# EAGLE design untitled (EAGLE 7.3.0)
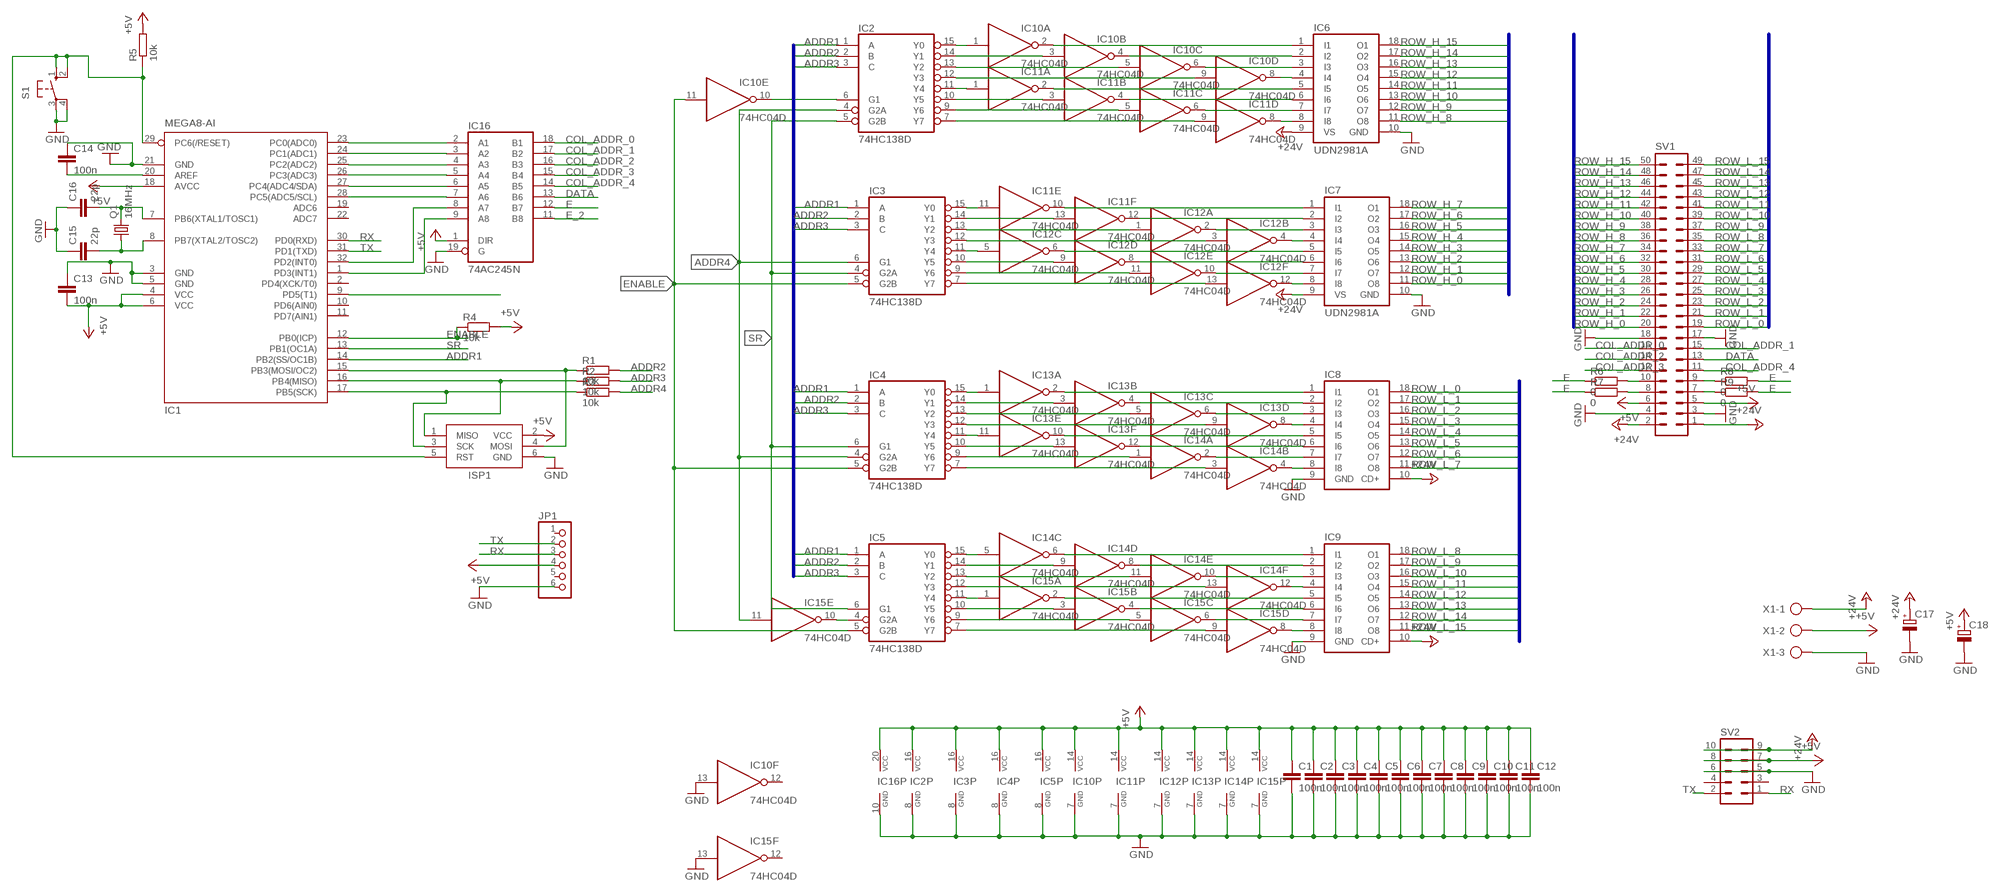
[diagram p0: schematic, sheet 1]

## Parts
C1  100n  C-EUC0805  [C0805]
C2  100n  C-EUC0805  [C0805]
C3  100n  C-EUC0805  [C0805]
C4  100n  C-EUC0805  [C0805]
C5  100n  C-EUC0805  [C0805]
C6  100n  C-EUC0805  [C0805]
C7  100n  C-EUC0805  [C0805]
C8  100n  C-EUC0805  [C0805]
C9  100n  C-EUC0805  [C0805]
C10  100n  C-EUC0805  [C0805]
C11  100n  C-EUC0805  [C0805]
C12  100n  C-EUC0805  [C0805]
C13  100n  C-EUC0805  [C0805]
C14  100n  C-EUC0805  [C0805]
C15  22p  C-EUC0805  [C0805]
C16  22p  C-EUC0805  [C0805]
C17  CPOL-EUTT5D7L  [TT5D7L]
C18  CPOL-EUTT2D7  [TT2D7]
IC1  MEGA8-AI  [TQFP32-08]
IC2  74HC138D  [SO16]
IC3  74HC138D  [SO16]
IC4  74HC138D  [SO16]
IC5  74HC138D  [SO16]
IC6  UDN2981A  [DIL18]
IC7  UDN2981A  [DIL18]
IC8  ULN2803A  [DIL18]
IC9  ULN2803A  [DIL18]
IC10  74HC04D  [SO14]
IC11  74HC04D  [SO14]
IC12  74HC04D  [SO14]
IC13  74HC04D  [SO14]
IC14  74HC04D  [SO14]
IC15  74HC04D  [SO14]
IC16  74AC245N  [DIL20]
ISP1  AVRISP-6  [AVRISP]
JP1  PINHD-1X6CB  [1X06-CLEANBIG]
Q1  16MHz  CRYSTALHC49UP  [HC49UP]
R1  10k  R-EU_R1206  [R1206]
R2  10k  R-EU_R1206  [R1206]
R3  10k  R-EU_R1206  [R1206]
R4  10k  R-EU_R1206  [R1206]
R5  10k  R-EU_R1206  [R1206]
R6  0  R-EU_M0805  [M0805]
R7  0  R-EU_M0805  [M0805]
R8  0  R-EU_M0805  [M0805]
R9  0  R-EU_M0805  [M0805]
S1  10-XX  [B3F-10XX]
SV1  ML50  [ML50]
SV2  ML10  [ML10]
X1  AK300/3  [AK300/3]

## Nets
+5V: C1.1 C2.1 C3.1 C4.1 C5.1 C6.1 C7.1 C8.1 C9.1 C10.1 C11.1 C12.1 C13.2 C18.+ IC1.4(VCC) IC1.6(VCC) IC1.18(AVCC) IC2.16(VCC) IC3.16(VCC) IC4.16(VCC) IC5.16(VCC) IC10.14(P:VCC) IC11.14(P:VCC) IC12.14(P:VCC) IC13.14(P:VCC) IC14.14(P:VCC) IC15.14(P:VCC) IC16.1(DIR) IC16.20(VCC) ISP1.2(VCC) JP1.4 R4.2 R5.2 SV1.5 SV1.6 SV2.7 SV2.8 X1.2
+24V: C17.+ IC6.9(VS) IC7.9(VS) IC8.10(CD+) IC9.10(CD+) SV1.1 SV1.2 SV2.9 SV2.10 X1.1
ADDR1: IC1.14(PB2(SS/OC1B)) IC2.1(A) IC3.1(A) IC4.1(A) IC5.1(A)
ADDR2: IC2.2(B) IC3.2(B) IC4.2(B) IC5.2(B) R1.2
ADDR3: IC2.3(C) IC3.3(C) IC4.3(C) IC5.3(C) R2.2
ADDR4: IC2.4(G2A) IC3.6(G1) IC4.4(G2A) IC15.11(E:I) R3.2
COL_ADDR_0: IC16.18(B1) SV1.16
COL_ADDR_1: IC16.17(B2) SV1.15
COL_ADDR_2: IC16.16(B3) SV1.14
COL_ADDR_3: IC16.15(B4) SV1.12
COL_ADDR_4: IC16.14(B5) SV1.11
DATA: IC16.13(B6) SV1.13
E: IC16.12(B7) R6.1 R7.1 R8.2 R9.2
E_2: IC16.11(B8)
ENABLE: IC1.12(PB0(ICP)) IC3.5(G2B) IC4.5(G2B) IC5.5(G2B) IC10.11(E:I) R4.1
GND: C1.2 C2.2 C3.2 C4.2 C5.2 C6.2 C7.2 C8.2 C9.2 C10.2 C11.2 C12.2 C13.1 C14.1 C15.1 C16.1 C17.- C18.- IC1.3(GND) IC1.5(GND) IC1.21(GND) IC2.8(GND) IC3.8(GND) IC4.8(GND) IC5.8(GND) IC6.10(GND) IC7.10(GND) IC8.9(GND) IC9.9(GND) IC10.7(P:GND) IC10.13(F:I) IC11.7(P:GND) IC12.7(P:GND) IC13.7(P:GND) IC14.7(P:GND) IC15.7(P:GND) IC15.13(F:I) IC16.10(GND) IC16.19(G) ISP1.6(GND) JP1.6 S1.3(P) S1.4(P1) SV1.3 SV1.4 SV1.17 SV1.18 SV2.5 SV2.6 X1.3
N$1: IC9.8(I8) IC15.8(D:O)
N$2: IC9.7(I7) IC15.6(C:O)
N$3: IC9.6(I6) IC15.4(B:O)
N$4: IC6.1(I1) IC10.2(A:O)
N$5: IC6.2(I2) IC10.4(B:O)
N$6: IC6.3(I3) IC10.6(C:O)
N$7: IC2.15(Y0) IC10.1(A:I)
N$8: IC2.14(Y1) IC10.3(B:I)
N$9: IC2.13(Y2) IC10.5(C:I)
N$10: IC5.10(Y5) IC15.3(B:I)
N$11: IC5.9(Y6) IC15.5(C:I)
N$12: IC5.7(Y7) IC15.9(D:I)
N$13: IC6.8(I8) IC11.8(D:O)
N$14: IC2.12(Y3) IC10.9(D:I)
N$15: IC2.11(Y4) IC11.1(A:I)
N$16: IC2.10(Y5) IC11.3(B:I)
N$17: IC2.9(Y6) IC11.5(C:I)
N$18: IC2.7(Y7) IC11.9(D:I)
N$19: IC6.7(I7) IC11.6(C:O)
N$20: IC6.6(I6) IC11.4(B:O)
N$21: IC6.5(I5) IC11.2(A:O)
N$22: IC6.4(I4) IC10.8(D:O)
N$23: IC7.1(I1) IC11.10(E:O)
N$24: IC7.2(I2) IC11.12(F:O)
N$25: IC7.3(I3) IC12.2(A:O)
N$26: IC3.15(Y0) IC11.11(E:I)
N$27: IC3.14(Y1) IC11.13(F:I)
N$28: IC3.13(Y2) IC12.1(A:I)
N$29: IC8.1(I1) IC13.2(A:O)
N$30: IC3.12(Y3) IC12.3(B:I)
N$31: IC3.11(Y4) IC12.5(C:I)
N$32: IC3.10(Y5) IC12.9(D:I)
N$33: IC3.9(Y6) IC12.11(E:I)
N$34: IC3.7(Y7) IC12.13(F:I)
N$35: IC7.7(I7) IC12.10(E:O)
N$36: IC7.6(I6) IC12.8(D:O)
N$37: IC7.5(I5) IC12.6(C:O)
N$38: IC8.2(I2) IC13.4(B:O)
N$39: IC8.3(I3) IC13.6(C:O)
N$40: IC4.15(Y0) IC13.1(A:I)
N$41: IC4.14(Y1) IC13.3(B:I)
N$42: IC4.13(Y2) IC13.5(C:I)
N$43: IC4.12(Y3) IC13.9(D:I)
N$44: IC4.11(Y4) IC13.11(E:I)
N$45: IC4.10(Y5) IC13.13(F:I)
N$46: IC4.9(Y6) IC14.1(A:I)
N$47: IC4.7(Y7) IC14.3(B:I)
N$48: IC8.7(I7) IC14.2(A:O)
N$49: IC8.6(I6) IC13.12(F:O)
N$50: IC8.5(I5) IC13.10(E:O)
N$51: IC7.4(I4) IC12.4(B:O)
N$52: IC7.8(I8) IC12.12(F:O)
N$53: IC8.4(I4) IC13.8(D:O)
N$54: IC8.8(I8) IC14.4(B:O)
N$55: IC5.11(Y4) IC15.1(A:I)
N$56: IC9.5(I5) IC15.2(A:O)
N$57: IC9.4(I4) IC14.12(F:O)
N$58: IC5.12(Y3) IC14.13(F:I)
N$59: IC5.13(Y2) IC14.11(E:I)
N$60: IC9.3(I3) IC14.10(E:O)
N$61: IC9.2(I2) IC14.8(D:O)
N$62: IC5.14(Y1) IC14.9(D:I)
N$63: IC5.15(Y0) IC14.5(C:I)
N$64: IC9.1(I1) IC14.6(C:O)
N$65: IC5.4(G2A) IC15.10(E:O)
N$66: IC1.15(PB3(MOSI/OC2)) ISP1.4(MOSI) R1.1
N$67: IC1.1(PD3(INT1)) IC16.9(A8)
N$69: IC1.16(PB4(MISO)) ISP1.1(MISO) R2.1
N$70: IC1.17(PB5(SCK)) ISP1.3(SCK) R3.1
N$71: IC1.32(PD2(INT0)) IC16.8(A7)
N$72: IC2.6(G1) IC10.10(E:O)
N$74: R6.2 SV1.10
N$75: IC1.9(PD5(T1))
N$76: IC1.23(PC0(ADC0)) IC16.2(A1)
N$77: IC1.24(PC1(ADC1)) IC16.3(A2)
N$78: IC1.25(PC2(ADC2)) IC16.4(A3)
N$79: IC1.26(PC3(ADC3)) IC16.5(A4)
N$80: IC1.27(PC4(ADC4/SDA)) IC16.6(A5)
N$81: IC1.28(PC5(ADC5/SCL)) IC16.7(A6)
N$82: C14.2 IC1.20(AREF)
N$83: IC1.29(PC6(/RESET)) ISP1.5(RST) R5.1 S1.1(S) S1.2(S1)
N$84: C16.2 IC1.7(PB6(XTAL1/TOSC1)) Q1.2
N$85: C15.2 IC1.8(PB7(XTAL2/TOSC2)) Q1.1
N$86: R7.2 SV1.8
N$87: R8.1 SV1.9
N$88: R9.1 SV1.7
ROW_H_0: IC7.11(O8) SV1.20
ROW_H_1: IC7.12(O7) SV1.22
ROW_H_2: IC7.13(O6) SV1.24
ROW_H_3: IC7.14(O5) SV1.26
ROW_H_4: IC7.15(O4) SV1.28
ROW_H_5: IC7.16(O3) SV1.30
ROW_H_6: IC7.17(O2) SV1.32
ROW_H_7: IC7.18(O1) SV1.34
ROW_H_8: IC6.11(O8) SV1.36
ROW_H_9: IC6.12(O7) SV1.38
ROW_H_10: IC6.13(O6) SV1.40
ROW_H_11: IC6.14(O5) SV1.42
ROW_H_12: IC6.15(O4) SV1.44
ROW_H_13: IC6.16(O3) SV1.46
ROW_H_14: IC6.17(O2) SV1.48
ROW_H_15: IC6.18(O1) SV1.50
ROW_L_0: IC8.18(O1) SV1.19
ROW_L_1: IC8.17(O2) SV1.21
ROW_L_2: IC8.16(O3) SV1.23
ROW_L_3: IC8.15(O4) SV1.25
ROW_L_4: IC8.14(O5) SV1.27
ROW_L_5: IC8.13(O6) SV1.29
ROW_L_6: IC8.12(O7) SV1.31
ROW_L_7: IC8.11(O8) SV1.33
ROW_L_8: IC9.18(O1) SV1.35
ROW_L_9: IC9.17(O2) SV1.37
ROW_L_10: IC9.16(O3) SV1.39
ROW_L_11: IC9.15(O4) SV1.41
ROW_L_12: IC9.14(O5) SV1.43
ROW_L_13: IC9.13(O6) SV1.45
ROW_L_14: IC9.12(O7) SV1.47
ROW_L_15: IC9.11(O8) SV1.49
RX: IC1.30(PD0(RXD)) JP1.3 SV2.1
SR: IC1.13(PB1(OC1A)) IC2.5(G2B) IC3.4(G2A) IC4.6(G1) IC5.6(G1)
TX: IC1.31(PD1(TXD)) JP1.2 SV2.2
Unconnected: IC1.2(PD4(XCK/T0)) IC1.10(PD6(AIN0)) IC1.11(PD7(AIN1)) IC1.19(ADC6) IC1.22(ADC7) IC10.12(F:O) IC15.12(F:O) JP1.1 JP1.5 SV2.3 SV2.4

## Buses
ROW_H_[0..15]
ROW_L_[0..15]
ADDR[1..3]

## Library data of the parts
C1-C16 = rcl:C-EU: CAPACITOR, European symbol
C17 C18 = rcl:CPOL-EU: POLARIZED CAPACITOR, European symbol
IC1 = atmel:MEGA8: MICROCONTROLLER 8 Kbytes FLASH, 1 kbytes SRAM, 512 bytes EEPROM, USART, 6-channel 10 bit ADC, 2-channel 8 bit ADC Pin compatible with Atmega48, ATMega88, ATMega168 Source: avr.lbr; MPN: ATMEGA8-16AU; OC_FARNELL: 9171371; OC_NEWARK: 73M8863
IC2-IC5 = 74xx-eu:74*138: 3-line to 8-line DECODER/DEMULTIPLEXER
IC6 IC7 = uln-udn:UDN298*: DRIVER ARRAY Source: Allegro Microsystems Inc. / UDN2981-UDN2984.pdf
IC8 IC9 = uln-udn:ULN2803A: DRIVER ARRAY
IC10-IC15 = 74xx-eu:74*04: Hex INVERTER
IC16 = 74xx-eu:74*245: Octal BUS TRANSCEIVER, 3-state
ISP1 = adafruit:AVRISP: AVR ISP HEADER Standard 6 pin header for AVR programming
JP1 = adafruit:PINHD-1X6: PIN HEADER
Q1 = crystal:CRYSTAL: CRYSTAL; OC_FARNELL: unknown; OC_NEWARK: unknown
R1-R9 = rcl:R-EU_: RESISTOR, European symbol
S1 = switch-omron:10-XX: OMRON SWITCH; MPN: B3F-1000; OC_FARNELL: 176432; OC_NEWARK: 36M3542
SV1 = con-harting-ml:ML50: HARTING; OC_FARNELL: unknown; OC_NEWARK: unknown
SV2 = con-harting-ml:ML10: HARTING; OC_FARNELL: unknown; OC_NEWARK: unknown
X1 = con-ptr500:AK300/3: CONNECTOR; OC_FARNELL: unknown; OC_NEWARK: unknown

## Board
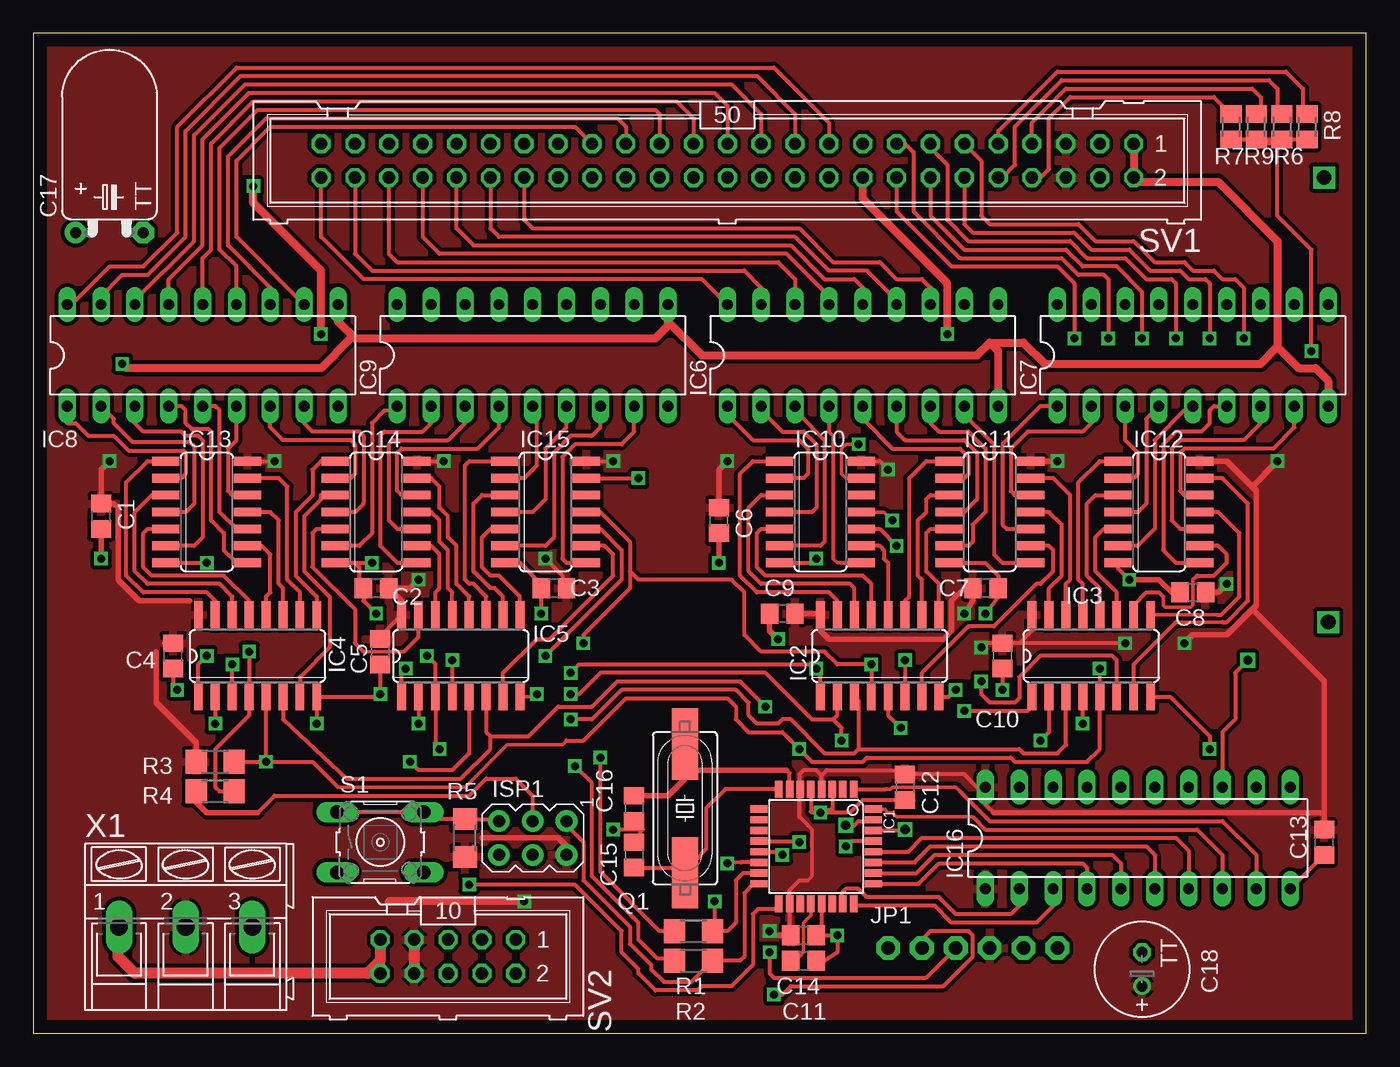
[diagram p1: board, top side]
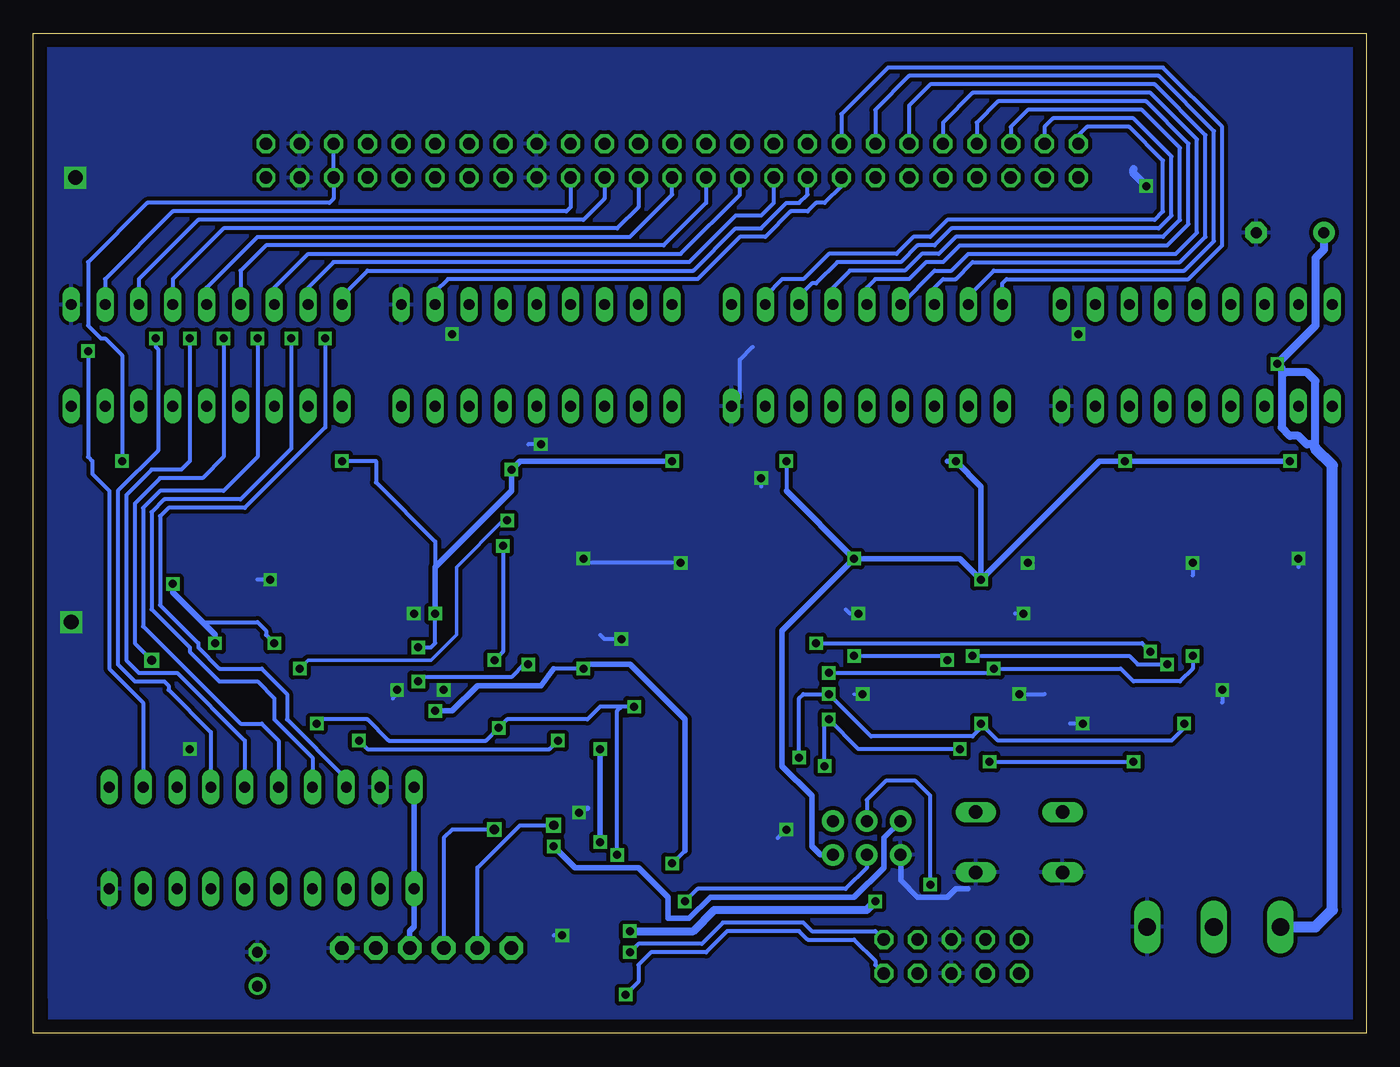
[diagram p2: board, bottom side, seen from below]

Size 100 x 75 mm. Coordinates in mm from the lower left corner, seen from the top.
Outline: 0,0 100,0 100,75 0,75 0,0
Copper layers (1*16): Top 0.035mm / dielectric 1.5mm / Bottom 0.035mm
Design rules "default *": minimum track width 6mil, minimum drill 10mil, track to track 8mil, track to pad 8mil, pad to pad 8mil, via to via 8mil, smd to smd 8mil, copper to edge 40mil, drill to drill 8mil, minimum pad ring 10mil, minimum via ring 8mil, stop-mask expansion 4mil, vias tented up to drill 0mil, thermal gap 10mil

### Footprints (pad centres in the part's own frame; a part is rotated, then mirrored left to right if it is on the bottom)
C0805 = smd 1.3 x 1.5: 1 -0.95,0; 2 0.95,0
TT5D7L = drill 0.813 pad 1.6: + -2.54,0 | drill 0.813 pad 1.6 octagon: - 2.54,0
TT2D7 = drill 0.813: + -1.27,0 | drill 0.813 octagon: - 1.27,0
TQFP32-08 = smd 1.27 x 0.559: 1 -4.293,2.8; 2 -4.293,2; 3 -4.293,1.2; 4 -4.293,0.4; 5 -4.293,-0.4; 6 -4.293,-1.2; 7 -4.293,-2; 8 -4.293,-2.8; 17 4.293,-2.8; 18 4.293,-2; 19 4.293,-1.2; 20 4.293,-0.4; 21 4.293,0.4; 22 4.293,1.2; 23 4.293,2; 24 4.293,2.8 | smd 0.559 x 1.27: 9 -2.8,-4.293; 10 -2,-4.293; 11 -1.2,-4.293; 12 -0.4,-4.293; 13 0.4,-4.293; 14 1.2,-4.293; 15 2,-4.293; 16 2.8,-4.293; 25 2.8,4.293; 26 2,4.293; 27 1.2,4.293; 28 0.4,4.293; 29 -0.4,4.293; 30 -1.2,4.293; 31 -2,4.293; 32 -2.8,4.293
SO16 = smd 0.66 x 2.032: 1 -4.445,-3.073; 2 -3.175,-3.073; 3 -1.905,-3.073; 4 -0.635,-3.073; 5 0.635,-3.073; 6 1.905,-3.073; 7 3.175,-3.073; 8 4.445,-3.073; 9 4.445,3.073; 10 3.175,3.073; 11 1.905,3.073; 12 0.635,3.073; 13 -0.635,3.073; 14 -1.905,3.073; 15 -3.175,3.073; 16 -4.445,3.073
DIL18 = drill 0.813 long: 1 -10.16,-3.81; 2 -7.62,-3.81; 3 -5.08,-3.81; 4 -2.54,-3.81; 5 0,-3.81; 6 2.54,-3.81; 7 5.08,-3.81; 8 7.62,-3.81; 9 10.16,-3.81; 10 10.16,3.81; 11 7.62,3.81; 12 5.08,3.81; 13 2.54,3.81; 14 0,3.81; 15 -2.54,3.81; 16 -5.08,3.81; 17 -7.62,3.81; 18 -10.16,3.81
SO14 = smd 0.66 x 2.032: 1 -3.81,-3.073; 2 -2.54,-3.073; 3 -1.27,-3.073; 4 0,-3.073; 5 1.27,-3.073; 6 2.54,-3.073; 7 3.81,-3.073; 8 3.81,3.073; 9 2.54,3.073; 10 1.27,3.073; 11 0,3.073; 12 -1.27,3.073; 13 -2.54,3.073; 14 -3.81,3.073
DIL20 = drill 0.813 long: 1 -11.43,-3.81; 2 -8.89,-3.81; 3 -6.35,-3.81; 4 -3.81,-3.81; 5 -1.27,-3.81; 6 1.27,-3.81; 7 3.81,-3.81; 8 6.35,-3.81; 9 8.89,-3.81; 10 11.43,-3.81; 11 11.43,3.81; 12 8.89,3.81; 13 6.35,3.81; 14 3.81,3.81; 15 1.27,3.81; 16 -1.27,3.81; 17 -3.81,3.81; 18 -6.35,3.81; 19 -8.89,3.81; 20 -11.43,3.81
AVRISP = drill 0.9 pad 1.626: 1 -1.27,2.54; 2 1.27,2.54; 3 -1.27,0; 4 1.27,0; 5 -1.27,-2.54; 6 1.27,-2.54
1X06-CLEANBIG = drill 1.016 pad 1.778 octagon: 1 -6.35,0; 2 -3.81,0; 3 -1.27,0; 4 1.27,0; 5 3.81,0; 6 6.35,0
HC49UP = smd 5.334 x 1.93: 1 -4.826,0; 2 4.826,0
R1206 = smd 1.6 x 1.803: 1 -1.422,0; 2 1.422,0
M0805 = smd 1.3 x 1.6: 1 -0.95,0; 2 0.95,0
B3F-10XX = drill 1.016 long: 1 -3.251,2.261; 2 3.251,2.261; 3 -3.251,-2.261; 4 3.251,-2.261
ML50 = drill 0.914 octagon: 1 -30.48,-1.27; 2 -30.48,1.27; 3 -27.94,-1.27; 4 -27.94,1.27; 5 -25.4,-1.27; 6 -25.4,1.27; 7 -22.86,-1.27; 8 -22.86,1.27; 9 -20.32,-1.27; 10 -20.32,1.27; 11 -17.78,-1.27; 12 -17.78,1.27; 13 -15.24,-1.27; 14 -15.24,1.27; 15 -12.7,-1.27; 16 -12.7,1.27; 17 -10.16,-1.27; 18 -10.16,1.27; 19 -7.62,-1.27; 20 -7.62,1.27; 21 -5.08,-1.27; 22 -5.08,1.27; 23 -2.54,-1.27; 24 -2.54,1.27; 25 0,-1.27; 26 0,1.27; 27 2.54,-1.27; 28 2.54,1.27; 29 5.08,-1.27; 30 5.08,1.27; 31 7.62,-1.27; 32 7.62,1.27; 33 10.16,-1.27; 34 10.16,1.27; 35 12.7,-1.27; 36 12.7,1.27; 37 15.24,-1.27; 38 15.24,1.27; 39 17.78,-1.27; 40 17.78,1.27; 41 20.32,-1.27; 42 20.32,1.27; 43 22.86,-1.27; 44 22.86,1.27; 45 25.4,-1.27; 46 25.4,1.27; 47 27.94,-1.27; 48 27.94,1.27; 49 30.48,-1.27; 50 30.48,1.27
ML10 = drill 0.914 octagon: 1 -5.08,-1.27; 2 -5.08,1.27; 3 -2.54,-1.27; 4 -2.54,1.27; 5 0,-1.27; 6 0,1.27; 7 2.54,-1.27; 8 2.54,1.27; 9 5.08,-1.27; 10 5.08,1.27
AK300/3 = drill 1.321 long: 1 -5.004,0; 2 0,0; 3 5.004,0

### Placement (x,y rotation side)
C1  5.08,38.78 270 top
C2  25.72,33.38 180 top
C3  39.05,33.38 180 top
C4  10.48,28.3 270 top
C5  26.04,28.62 270 top
C6  51.44,38.47 270 top
C7  71.44,33.38 0 top
C8  87,33.07 180 top
C9  56.2,31.48 180 top
C10  72.71,28.3 270 top
C11  57.78,7.35 0 top
C12  65.41,18.46 270 top
C13  96.84,14.34 90 top
C14  57.78,5.45 180 top
C15  45.09,13.38 270 top
C16  45.09,16.88 90 top
C17  5.71,60.05 0 top
C18  83.19,4.81 90 top
IC1  58.74,14.02 270 top
IC2  63.5,28.3 0 top
IC3  79.38,28.3 0 top
IC4  16.83,28.3 0 top
IC5  32.07,28.3 0 top
IC6  62.23,50.85 0 top
IC7  87,50.85 0 top
IC8  12.7,50.85 0 top
IC9  37.47,50.85 0 top
IC10  59.05,39.1 270 top
IC11  71.75,39.1 270 top
IC12  84.45,39.1 270 top
IC13  13.02,39.1 270 top
IC14  25.72,39.1 270 top
IC15  38.42,39.1 270 top
IC16  82.87,14.65 0 top
ISP1  37.47,14.65 270 top
JP1  70.48,6.4 0 top
Q1  48.9,16.88 90 top
R1  49.53,7.67 180 top
R2  49.53,5.45 180 top
R3  13.65,18.14 0 top
R4  13.65,20.37 180 top
R5  32.38,14.65 270 top
R6  93.66,67.99 90 top
R7  89.85,67.99 90 top
R8  95.57,67.99 270 top
R9  91.76,67.99 270 top
S1  26.04,14.34 0 top
SV1  52.07,65.45 180 top
SV2  31.11,5.76 180 top
X1  11.43,7.99 0 top

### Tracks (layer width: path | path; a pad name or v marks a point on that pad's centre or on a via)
+5V  (via drill 0.6)
  Top 0.254: 58.1,15.61 58.42,15.29 58.42,11.79 58.1,11.48
  Top 0.305: IC13.14 v18.1,42.91 | IC14.14 v30.8,42.91 | 70.49,32.44 C7.1 69.85,33.38 | 73.98,29.26 73.03,29.26 | 73.03,29.26 C10.1 | IC3.16 74.93,30.21 73.98,29.26 | 73.03,29.26 71.44,29.26 v71.12,28.94 | IC10.14 63.5,42.91 v64.14,42.27 | IC15.14 v43.5,42.91 | v38.42,35.61 39.69,34.34 39.69,33.7 C3.1 | C5.1 26.04,29.79 IC5.16 | IC4.16 12.38,31.8 | v81.92,29.26 73.98,29.26 | 58.95,31.48 IC2.16 | 72.07,16.56 71.44,17.19 IC16.20 70.8,18.46 69.85,19.41 C12.1 | 96.52,16.56 96.84,16.24 | IC1.4 59.14,19.33 | 59.14,19.33 58.74,19.73 57.78,19.73 57.47,19.41 57.47,18.38 IC1.6 57.47,18.24 57.47,16.24 58.1,15.61 | C12.1 65.09,19.09 | 59.14,19.33 59.54,19.73 65.08,19.73 C12.1 | C11.1 56.74,7.76 IC1.18 56.74,10.75 57.47,11.48 58.1,11.48 | R5.2 32.38,13.38 33.02,14.02 | 65.41,19.1 C12.1 | 56.83,7.03 57.15,7.35
  Top 0.406: 70.49,32.44 v69.85,31.48 | C8.1 88.9,33.07 v89.53,33.7 | IC2.16 59.05,30.21 59.69,29.57 68.26,29.57 68.9,30.21 68.9,32.43 69.85,33.38 | C6.1 51.44,42.27 v52.07,42.91 | IC5.16 27.62,32.43 C2.1 28.26,33.38 v28.89,34.02 | v5.71,42.91 5.08,42.27 C1.1 5.4,39.73 6.03,39.73 6.35,39.42 6.35,34.02 7.94,32.43 11.75,32.43 | IC11.14 v76.83,42.91 | C9.1 58.95,31.48 | 91.44,41.01 89.53,42.91 IC12.14 | 91.44,41.01 91.76,40.69 91.76,32.11 91.44,31.8 | 91.44,31.8 89.53,29.89 87,29.89 v86.36,29.26 | v93.34,42.91 91.44,41.01 | C13.2 96.84,16.24 96.84,26.4 91.44,31.8 | 72.07,16.56 96.52,16.56 | R4.2 12.23,21.79 9.21,24.81 9.21,28.62 | 9.84,29.26 C4.1 | 33.66,14.65 39.37,14.65 40.01,14.02 ISP1.2 | 57.15,7.35 55.56,7.35 v55.24,7.67
  Top 0.61: v36.83,9.89 26.67,9.89
  Top 0.813: SV2.7 SV2.8
  Bottom 0.305: v71.12,28.94 70.17,28.94 69.85,29.26 v69.85,31.48 | v89.53,33.7 89.53,33.07 | v43.5,42.91 43.5,40.69 | 69.85,34.97 69.85,36.88 74.3,41.32 74.3,42.91 v76.83,42.91 | 87.31,30.84 83.19,30.84 82.55,30.21 82.55,29.89 v81.92,29.26 | SV1.5 SV1.6 77.47,62.59 77.79,62.28 91.44,62.28 95.89,57.83 95.89,53.07 94.93,52.12 94.61,52.12 93.34,50.85 v93.34,42.91 | v38.42,35.61 39.69,34.34
  Bottom 0.406: 31.43,42.91 v30.8,42.91 28.89,41.01 v28.89,34.02 | v69.85,31.48 69.85,34.97 64.14,40.69 v64.14,42.27 63.5,42.91 v52.07,42.91 | 43.5,40.69 v38.42,35.61 | v5.71,42.91 v18.1,42.91 20,42.91 v28.89,34.02 | v38.42,35.61 30.48,35.61 v28.89,34.02 | 89.53,33.07 87.31,30.84 86.36,29.89 v86.36,29.26 | IC16.20 IC16.1 71.44,7.99 71.75,7.67 JP1.4 | v38.42,35.61 43.81,30.21 43.81,20.05 41.59,17.83 41.59,14.02 40.96,13.38 ISP1.2
  Bottom 0.61: v55.24,7.67 50.48,7.67 48.9,9.26 37.47,9.26 v36.83,9.89
  pour Top (isolate 0.305): -0.68,-2.68 102.42,-4.68 101.42,77.34 -4.68,78.34
+24V  (via drill 0.6)
  Top 0.61: SV1.1 SV1.2 82.87,63.87 88.9,63.87 93.34,59.42 93.34,51.48 | 93.34,51.48 94.93,49.9 96.2,49.9 97.16,48.94 IC7.9 | IC8.10 22.86,53.39 24.13,52.12 | 24.13,52.12 46.67,52.12 47.62,53.07 47.62,53.39 | 47.62,53.39 IC9.10 | IC6.9 72.39,51.16 71.75,51.8 | 47.62,53.39 50.16,50.85 70.8,50.85 71.75,51.8 | 71.75,51.8 74.3,51.8 75.88,50.21 92.08,50.21 93.34,51.48 | SV2.10 SV2.9 | 24.13,52.12 23.81,52.12 21.59,49.9 6.99,49.9 v6.67,50.21
  Top 0.813: SV2.9 26.04,5.45 25.08,4.49 7.62,4.49 6.35,5.76 6.35,7.91 X1.1
  Bottom 0.61: 6.03,49.58 4.45,49.58 3.81,48.94 3.81,43.86 4.13,44.18 4.45,44.18 5.08,44.81 5.71,44.81 6.35,45.45 6.35,49.9 v6.67,50.21 3.81,53.07 3.81,58.15 3.17,58.78 C17.+
  Bottom 0.813: X1.1 3.81,7.99 2.54,9.26 2.54,42.59 3.81,43.86
ADDR1  (via drill 0.6)
  Top 0.305: IC5.1 27.62,27.04 v27.94,27.35 | v40.32,27.04 40.96,27.67 58.42,27.67 v58.74,27.35 59.05,26.72 IC2.1 | v69.85,24.18 74.61,24.18 74.93,24.5 IC3.1 | IC4.1 12.38,27.67 v13.02,28.3 | IC1.14 53.09,12.82 v52.07,12.75
  Bottom 0.305: v13.02,28.3 13.02,27.35 13.97,26.4 17.46,26.4 18.41,27.35 v27.94,27.35 28.26,27.04 v40.32,27.04 | v58.74,27.35 60.96,27.35 | v52.07,12.75 52.07,13.06 51.75,13.06 51.12,13.7
  Bottom 0.406: 60.96,27.35 61.91,26.08 66.67,26.08 68.58,24.18 v69.85,24.18 | v58.74,27.35 58.42,27.67 55.24,27.67 51.12,23.54 51.12,13.7
ADDR2  (via drill 0.6)
  Top 0.305: IC5.2 v28.89,23.23 | 60.01,23.54 58.42,23.54 54.93,27.04 42.55,27.04 40.96,25.45 v40.32,25.45 | 60.01,23.54 60.33,23.86 IC2.2 | IC3.2 76.2,22.59 v75.56,21.95 | IC4.2 v13.65,23.23 | v60.64,21.95 60.64,22.91 60.01,23.54 | R1.2 46.99,7.67 42.55,12.11 v42.55,20.68
  Bottom 0.305: v13.65,23.23 13.65,22.91 14.61,21.95 27.62,21.95 v28.89,23.23 28.89,22.91 29.53,22.27 37.15,22.27 v40.32,25.45 42.23,25.45 42.55,25.13 v42.55,20.68 | v75.56,21.95 74.93,21.32 61.28,21.32 v60.64,21.95
ADDR3  (via drill 0.6)
  Top 0.305: v29.53,28.3 30.16,27.67 IC5.3 30.16,21.64 v30.48,21.32 | IC4.3 v14.92,27.67 | 61.91,21.32 61.59,21 59.37,21 56.83,23.54 56.2,23.54 55.88,23.23 54.29,23.23 53.66,23.86 53.66,24.81 52.7,25.77 44.13,25.77 41.91,23.54 v40.32,23.54 | IC2.3 61.91,24.91 61.91,21.32 | IC3.3 77.47,21.64 76.83,21 74.3,21 73.98,21.32 61.91,21.32 | R2.2 48.11,5.6 46.84,5.6 45.4,7.03 45.4,8.3 41.91,11.79 41.91,18.78 v40.64,20.05
  Bottom 0.305: v29.53,28.3 17.78,28.3 17.14,27.67 v14.92,27.67 | v30.48,21.32 38.1,21.32 v40.32,23.54 40.64,23.23 v40.64,20.05
ADDR4  (via drill 0.6)
  Top 0.305: IC15.11 42.55,39.1 44.77,36.88 44.77,34.66 | 44.77,34.66 44.77,33.38 41.27,29.89 v41.27,29.26 | v16.19,28.62 IC4.4 16.19,23.86 13.65,21.32 13.65,18.46 13.97,18.14 R3.2 | IC3.6 81.28,27.99 80.96,28.3 75.56,28.3 73.98,26.72 73.98,25.13 73.66,24.81 71.75,24.81 71.12,25.45 v71.12,26.4 | IC2.4 v62.87,27.67 60.33,27.67 59.37,28.62 54.61,28.62 53.34,29.89 53.34,33.07 52.39,34.02 45.4,34.02 44.77,34.66
  Bottom 0.305: v41.27,29.26 16.83,29.26 v16.19,28.62 | v62.87,27.67 63.18,27.67 64.14,26.72 70.8,26.72 v71.12,26.4
COL_ADDR_0  (via drill 0.6)
  Top 0.305: SV1.16 64.77,61.64 68.9,57.52 76.83,57.52 78.11,56.24 v78.11,52.12
  Bottom 0.305: v78.11,52.12 78.11,45.45 84.14,39.42 89.85,39.42 90.49,38.78 90.49,32.11 87.63,29.26 87.63,28.94 86.04,27.35 82.87,27.35 80.96,25.45 80.96,23.54 76.52,19.1 IC16.18
COL_ADDR_1  (via drill 0.6)
  Top 0.305: SV1.15 65.41,66.72 66.04,66.09 66.04,61.64 69.53,58.15 77.15,58.15 78.42,56.88 80.33,56.88 80.64,56.56 v80.64,52.12
  Bottom 0.305: v80.64,52.12 80.64,43.86 84.45,40.05 90.17,40.05 91.12,39.1 91.12,31.8 88.27,28.94 88.27,28.62 86.04,26.4 83.19,26.4 81.92,25.13 81.92,23.54 79.06,20.68 IC16.17
COL_ADDR_2  (via drill 0.6)
  Top 0.305: SV1.14 67.31,61.33 69.85,58.78 77.47,58.78 78.74,57.52 81.28,57.52 83.19,55.61 v83.19,52.12
  Bottom 0.305: v83.19,52.12 83.19,43.23 85.72,40.69 90.49,40.69 91.76,39.42 91.76,30.53 84.45,23.23 82.87,23.23 81.6,21.95 IC16.16
COL_ADDR_3  (via drill 0.6)
  Top 0.305: SV1.12 69.85,60.69 70.48,60.05 78.11,60.05 79.38,58.78 82.23,58.78 83.82,57.2 86.04,57.2 86.68,56.56 87.95,56.56 88.27,56.24 v88.27,52.12
  Bottom 0.305: v88.27,52.12 88.27,42.91 88.9,42.27 91.12,42.27 93.03,40.37 93.03,27.99 92.08,27.04 89.22,27.04 84.14,21.95 IC16.15
COL_ADDR_4  (via drill 0.6)
  Top 0.305: SV1.11 71.12,65.45 71.12,61.33 71.75,60.69 78.42,60.69 79.69,59.42 82.55,59.42 84.14,57.83 86.36,57.83 87,57.2 88.58,57.2 89.22,56.56 90.17,56.56 90.81,55.93 v90.81,52.12
  Bottom 0.305: v90.81,52.12 90.81,51.48 90.65,51.32 90.65,43.7 93.66,40.69 93.66,27.67 92.39,26.4 90.17,26.4 89.85,26.08 89.85,25.77 86.68,22.59 IC16.14
DATA  (via drill 0.6, 0.7)
  Top 0.305: SV1.13 67.31,66.41 68.58,65.14 68.58,61.01 70.17,59.42 77.79,59.42 79.06,58.15 81.92,58.15 83.5,56.56 85.41,56.56 85.72,56.24 v85.72,52.12 | v91.12,27.99 90.17,27.04 90.17,23.54 89.22,22.59 IC16.13
  Bottom 0.305: v85.72,52.12 85.72,43.23 87.31,41.64 90.49,41.64 92.39,39.73 92.39,29.26 v91.12,27.99
E  (via drill 0.6)
  Top 0.305: R7.1 R9.2 | R9.2 R6.1 | R6.1 R8.2 | v95.89,51.16 95.89,58.78 93.34,61.33 93.34,66.72 | 93.34,66.72 R6.1 | 93.34,66.72 92.08,66.72 R9.2
  Bottom 0.305: IC16.12 91.76,24.81 94.3,27.35 94.3,40.69 95.57,41.96 95.57,42.91 95.89,43.23 v95.89,51.16
ENABLE  (via drill 0.6)
  Top 0.254: IC10.11 63.82,39.1 v64.45,38.47 | v80.01,27.35 IC3.5 | 22.86,18.46 32.38,18.46 35.56,21.64 39.69,21.64 40.01,21.95
  Top 0.305: v17.46,20.37 IC4.5 | IC5.5 32.7,21 31.43,19.73 28.89,19.73 v28.26,20.37 | v17.46,20.37 20.95,20.37 22.86,18.46 | IC3.5 80.01,21.32 79.06,20.37 73.66,20.37 73.34,20.68 62.55,20.68 62.23,20.37 58.42,20.37 v57.47,21.32 56.2,22.59 53.66,22.59 52.7,23.54 52.7,24.5 52.07,25.13 44.45,25.13 41.27,21.95 40.01,21.95 | IC1.12 57.38,14.42 v57.47,14.34 | R4.1 v17.46,20.37
  Bottom 0.254: v64.45,38.47 64.77,38.47 68.26,34.97 68.26,29.89 70.17,27.99 79.38,27.99 v80.01,27.35
  Bottom 0.305: v28.26,20.37 v17.46,20.37
  Bottom 0.406: v57.47,14.34 v57.47,21.32
GND  (via drill 0.6, 1.1 pad 0.81)
  Top 0.254: v61.91,44.18 60.96,44.18 60.64,43.86 60.64,41.96 60.96,41.64 IC10.13 | IC5.8 37.57,25.23 v37.78,25.45
  Top 0.305: IC13.7 v13.02,35.29 | IC15.7 36.51,35.29 38.1,33.7 C3.2 v38.1,31.48 | v25.4,35.29 IC14.7 24.13,35.29 24.45,34.97 24.45,33.7 C2.2 24.77,32.43 v25.72,31.48 | IC11.7 71.44,35.29 72.39,34.34 C7.2 72.39,32.75 v71.44,31.48 | IC12.7 81.38,34.87 v82.23,34.02 | C8.2 85.41,33.07 | IC3.8 85.31,25.23 88.27,22.27 v88.27,21.32 | IC2.8 68.68,25.23 v69.22,25.77 | C10.2 v72.71,25.77 | IC10.7 58.42,35.29 v58.74,35.61 | C5.2 v26.04,25.45 25.82,25.23 IC4.8 v21.27,23.23 | IC15.13 v45.4,41.64 | C4.2 10.48,26.08 v10.79,25.77 | C13.1 IC16.10 | IC1.3 59.94,16.8 v59.05,16.56 | IC1.5 58.34,16.64 58.42,16.56 v59.05,16.56 | v59.05,16.56 61.28,16.56 62.23,17.51 C12.2 | 45.72,15.29 C16.1 | C15.1 45.72,15.29 | 45.72,15.29 v43.5,15.29 | IC1.21 59.14,8.07 C11.2 v60.33,7.35 60.33,6.08 59.37,5.45 C14.1 | 66.04,17.51 C12.2 | C12.2
  Top 0.406: 85.41,33.07 84.45,34.02 v82.23,34.02 | C6.2 v51.44,35.29 | C1.2 v5.08,35.61 | C9.2 55.25,30.21 v55.88,29.57
  Top 0.61: v21.59,52.44 21.59,57.2 16.51,62.28 v16.51,63.55 | v68.58,52.44 68.58,56.24 62.23,62.59 SV1.18
  Bottom 0.254: v37.78,25.45 38.42,25.45
  Bottom 0.305: v13.02,35.29 13.02,34.34 | v38.1,31.48 38.73,31.48 39.05,31.8 | v25.4,35.29 25.72,34.97 | v71.44,31.48 71.12,31.48 | v82.23,34.02 83.19,34.02 | v72.71,25.77 72.71,25.45 73.03,25.13 | 59.05,35.29 v58.74,35.61 58.42,35.29 v51.44,35.29 | v25.72,31.48 26.35,31.48 | v26.04,25.45 24.13,25.45 | v21.27,23.23 22.23,23.23 | v5.08,35.61 5.08,34.97 | v61.91,44.18 62.87,44.18 | v55.88,29.57 57.15,29.57 57.47,29.89 | v45.4,41.64 45.4,41.01 | v10.79,25.77 10.79,24.81 | IC9.9 46.99,47.67 46.99,50.53 46.04,51.48 | v43.5,15.29 44.13,14.65 | v60.33,7.35 60.96,7.35
  Bottom 0.406: v59.05,16.56 58.42,16.88 | ISP1.6 34.92,11.48 33.66,10.21 31.43,10.21 30.8,10.84 29.88,10.84
  Bottom 0.61: v16.51,63.55 17.46,64.5 17.46,64.82
  other vias: 96.84,64.18 97.16,30.84
  pour Bottom (isolate 0.305): -1.36,-4.37 98.74,-0.36 99.38,101.01 0,101.33
N$1
  Top 0.305: IC15.8 40.01,35.29 39.69,35.61 39.69,43.23 40.64,44.18 44.13,44.18 45.09,45.13 IC9.8
N$2
  Top 0.305: IC15.6 38.42,36.56 39.05,37.2 39.05,43.55 40.32,44.81 41.91,44.81 42.55,45.45 IC9.7
N$3
  Top 0.305: IC15.4 37.47,39.1 38.42,40.05 38.42,43.86 40.01,45.45 IC9.6
N$4
  Top 0.305: IC6.1 52.07,46.4 53.98,44.5 57.47,44.5 58.1,43.86 58.1,41.96 57.78,41.64 IC10.2
N$5
  Top 0.305: IC6.2 54.61,46.72 56.2,45.13 57.78,45.13 58.74,44.18 58.74,39.42 58.42,39.1 IC10.4
N$6
  Top 0.305: IC6.3 57.15,46.4 57.47,46.4 59.37,44.5 59.37,36.88 59.05,36.56 IC10.6
N$7
  Top 0.305: IC2.15 60.33,32.43 59.69,33.07 54.29,33.07 53.02,34.34 53.02,41.96 53.98,42.91 IC10.1
N$8
  Top 0.305: IC2.14 61.59,33.38 61.28,33.7 54.61,33.7 53.66,34.66 53.66,39.42 54.61,40.37 IC10.3
N$9
  Top 0.305: IC2.13 62.87,33.7 62.23,34.34 54.93,34.34 54.29,34.97 54.29,37.51 54.61,37.83 IC10.5
N$10
  Top 0.305: IC5.10 35.24,32.75 34.61,33.38 34.29,33.38 33.02,34.66 33.02,39.73 33.66,40.37 IC15.3
N$11
  Top 0.305: IC5.9 36.51,32.75 34.92,34.34 34.29,34.34 33.66,34.97 33.66,37.2 34.29,37.83 IC15.5
N$12
  Top 0.305: IC5.7 35.24,27.04 37.78,29.57 38.73,29.57 43.5,34.34 43.5,35.92 42.86,36.56 IC15.9
N$13
  Top 0.305: IC6.8 69.85,46.4 72.07,44.18 72.07,35.92 72.71,35.29 IC11.8
N$14
  Top 0.305: IC10.9 63.5,36.56 63.82,36.24 63.82,35.61 64.14,35.29 IC2.12
N$15
  Top 0.305: IC2.11 65.41,32.43 65.72,32.75 65.72,41.64 66.99,42.91 IC11.1
N$16
  Top 0.305: IC2.10 66.67,34.02 66.36,34.34 66.36,38.47 66.99,39.1 66.99,40.05 67.31,40.37 IC11.3
N$17
  Top 0.305: IC2.9 67.94,33.7 66.99,34.66 66.99,37.51 67.31,37.83 IC11.5 69.53,37.83
N$18
  Top 0.305: IC2.7 66.67,27.04 70.17,30.53 72.07,30.53 75.25,33.7 75.56,33.7 76.52,34.66 76.52,36.24 76.2,36.56 IC11.9
N$19
  Top 0.305: IC6.7 67.31,45.77 67.94,45.13 70.17,45.13 71.44,43.86 71.44,39.1 70.48,38.15 70.48,36.88 70.17,36.56 IC11.6
N$20
  Top 0.305: IC6.6 64.77,45.13 65.41,44.5 69.85,44.5 70.8,43.55 70.8,40.05 69.85,39.1 IC11.4
N$21
  Top 0.305: IC6.5 62.23,46.09 64.45,43.86 69.53,43.86 70.17,43.23 70.17,41.96 69.85,41.64 IC11.2
N$22
  Top 0.254: 60.64,35.29 60.33,35.29 60.01,35.61 | 60.01,44.5 60.01,44.81 59.69,45.13
  Top 0.305: IC6.4 59.69,45.13 | 60.01,44.5 60.01,35.61 | 60.64,35.29 IC10.8
N$23
  Top 0.305: IC11.10 73.03,37.83 72.71,38.15 72.71,44.18 75.56,47.04 IC7.1
N$24
  Top 0.305: IC11.12 73.66,40.37 73.34,40.69 73.34,43.86 74.61,45.13 78.74,45.13 79.38,45.77 IC7.2
N$25
  Top 0.305: IC12.2 82.55,41.64 82.87,41.96 82.87,43.55 81.92,44.5 IC7.3
N$26
  Top 0.305: IC3.15 76.2,33.38 77.15,34.34 77.15,38.15 76.2,39.1 IC11.11
N$27
  Top 0.305: IC3.14 77.47,33.7 77.79,34.02 77.79,40.37 76.52,41.64 IC11.13
N$28
  Top 0.305: IC3.13 78.74,33.7 78.42,34.02 78.42,41.32 80.01,42.91 IC12.1
N$29
  Top 0.305: IC13.2 11.11,41.64 11.43,41.96 11.43,43.55 11.27,43.7 7.14,43.7 6.03,44.81 4.13,44.81 3.17,45.77 2.54,45.77 IC8.1
N$30
  Top 0.305: IC3.12 80.01,33.38 79.06,34.34 79.06,39.73 79.69,40.37 IC12.3
N$31
  Top 0.305: IC3.11 81.28,33.07 79.69,34.66 79.69,37.2 80.33,37.83 IC12.5
N$32
  Top 0.254: 84.77,32.75 84.77,32.11 84.93,31.96 86.84,31.96 87,32.11 87,34.02
  Top 0.305: IC3.10 82.55,32.11 83.5,33.07 84.45,33.07 84.77,32.75 | 87,34.02 87.31,34.34 88.58,34.34 89.53,35.29 89.53,35.92 88.9,36.56 IC12.9
N$33
  Top 0.254: IC3.9 88.8,31.38
  Top 0.305: IC12.11 88.9,39.1 90.49,37.51 90.49,32.75 89.12,31.38 88.8,31.38
N$34
  Top 0.254: 85.72,30.84 89.22,30.84
  Top 0.305: IC3.7 82.55,27.67 85.72,30.84 | IC12.13 89.22,41.64 91.12,39.73 91.12,32.43 89.53,30.84 89.22,30.84
N$35
  Top 0.305: IC7.7 92.08,45.77 90.81,44.5 86.04,44.5 85.41,43.86 85.41,38.47 86.04,37.83 IC12.10
N$36
  Top 0.305: IC12.8 85.72,35.29 84.77,36.24 84.77,44.18 85.72,45.13 87.63,45.13 88.27,45.77 88.27,46.72 88.58,47.04 IC7.6
N$37
  Top 0.305: IC12.6 82.87,36.56 84.14,37.83 84.14,44.5 86.36,46.72 86.68,46.72 IC7.5
N$38
  Top 0.305: 9.53,39.1 IC13.4 11.43,39.1 12.06,39.73 12.06,44.02 11.75,44.34 7.46,44.34 6.03,45.77 6.03,46.09 IC8.2
N$39
  Top 0.305: IC13.6 12.06,36.56 12.7,37.2 12.7,44.5 12.38,44.81 11.43,44.81 11.11,45.13 8.26,45.13 7.62,45.77 IC8.3
N$40
  Top 0.305: IC4.15 13.65,32.43 13.02,33.07 8.26,33.07 6.99,34.34 6.99,41.32 8.57,42.91 IC13.1 10.48,42.91
N$41
  Top 0.305: IC4.14 14.92,32.75 13.97,33.7 8.57,33.7 7.62,34.66 7.62,39.1 8.89,40.37 IC13.3 10.48,40.37
N$42
  Top 0.305: IC4.13 16.19,32.43 14.29,34.34 8.89,34.34 8.26,34.97 8.26,37.51 8.57,37.83 IC13.5
N$43
  Top 0.305: IC4.12 17.46,32.75 17.78,33.07 17.78,35.92 17.14,36.56 IC13.9
N$44
  Top 0.305: IC4.11 18.73,33.38 18.41,33.7 18.41,38.47 17.78,39.1 IC13.11
N$45
  Top 0.305: IC4.10 20,33.07 19.05,34.02 19.05,41.01 18.41,41.64 IC13.13
N$46
  Top 0.305: IC14.1 21.59,42.91 20.95,42.27 20.95,40.37 19.68,39.1 19.68,34.34 21.27,32.75 IC4.9
N$47
  Top 0.305: 22.23,40.37 IC14.3 21.59,40.37 21.59,40.05 20.32,38.78 20.32,34.66 22.23,32.75 22.23,28.94 20,26.72 IC4.7
N$48
  Top 0.305: IC14.2 23.81,41.64 24.13,41.96 24.13,44.18 23.81,44.5 18.73,44.5 17.78,45.45 IC8.7
N$49
  Top 0.305: IC13.12 14.92,40.37 14.61,40.69 14.61,43.86 15.24,44.5 IC8.6
N$50
  Top 0.305: IC13.10 15.24,37.83 13.97,39.1 13.97,46.72 13.65,47.04 IC8.5
N$51
  Top 0.305: IC12.4 82.87,39.1 83.5,39.73 83.5,46.09 IC7.4
N$52
  Top 0.305: IC12.12 86.36,40.37 86.04,40.69 86.04,43.55 86.36,43.86 93.03,43.86 94.61,45.45 IC7.8
N$53
  Top 0.305: IC13.8 15.24,35.29 14.29,36.24 14.29,37.51 13.34,38.47 13.34,45.13 13.18,45.29 11.91,45.29 11.43,45.77 11.43,46.72 11.11,47.04 IC8.4
N$54
  Top 0.305: IC14.4 24.13,39.1 24.77,39.73 24.77,44.81 24.45,45.13 20.95,45.13 20.32,45.77 IC8.8
N$55
  Top 0.305: IC5.11 33.97,32.75 33.02,33.7 32.7,33.7 32.38,34.02 32.38,42.59 32.7,42.91 IC15.1
N$56
  Top 0.305: IC15.2 36.83,41.64 37.78,42.59 37.78,46.72 IC9.5
N$57
  Top 0.305: IC14.12 27.62,40.37 27.3,40.69 27.3,43.55 27.62,43.86 33.34,43.86 34.92,45.45 IC9.4
N$58
  Top 0.305: IC5.12 32.7,32.75 31.75,33.7 31.75,36.56 31.11,37.2 31.11,38.78 30.48,39.42 30.48,41.01 29.84,41.64 IC14.13
N$59
  Top 0.305: IC5.13 31.43,33.07 31.11,33.38 31.11,36.24 30.48,36.88 30.48,38.47 29.84,39.1 IC14.11
N$60
  Top 0.305: IC14.10 27.3,37.83 26.67,38.47 26.67,44.18 26.99,44.5 31.11,44.5 32.38,45.77 IC9.3 32.38,47.67
N$61
  Top 0.305: IC14.8 27.3,35.29 26.04,36.56 26.04,44.81 26.35,45.13 29.21,45.13 29.84,45.77 IC9.2
N$62
  Top 0.305: IC5.14 30.16,33.07 30.48,33.38 30.48,35.92 29.84,36.56 IC14.9
N$63
  Top 0.254: 24.77,28.62 27.78,28.62
  Top 0.305: IC14.5 21.27,37.83 20.95,37.51 20.95,34.97 24.13,31.8 24.13,29.26 24.77,28.62 | 27.78,28.62 28.89,29.73 IC5.15
N$64
  Top 0.305: IC14.6 24.45,36.56 25.4,37.51 25.4,45.77 26.35,46.72 26.99,46.72 IC9.1
N$65  (via drill 0.6)
  Top 0.305: IC15.10 42.55,37.83 44.13,36.24 44.13,34.02 v38.42,28.3 | v31.43,27.99 IC5.4
  Bottom 0.305: v38.42,28.3 31.75,28.3 v31.43,27.99
N$66  (via drill 0.6)
  Top 0.305: IC1.15 53.24,12.02 52.7,11.48 52.7,8.3 52.07,7.67 R1.1 51.12,7.83 v51.12,9.89
  Bottom 0.305: ISP1.4 37.47,12.43 39.05,10.84 50.16,10.84 v51.12,9.89
N$67
  Top 0.254: 63.97,18.31 64.3,18.31 64.45,18.46 69.22,18.46 69.53,18.14
  Top 0.305: IC1.1 63.97,18.31 | 69.53,18.14 71.75,15.92 89.22,15.92 91.76,13.38 IC16.9
N$69
  Top 0.305: ISP1.1 40.01,15.61 41.27,14.34 41.27,11.48 44.77,7.99 44.77,6.71 46.35,5.13 46.35,4.81 47.31,3.86 49.36,3.86 R2.1 53.02,5.45 53.34,5.76 53.34,10.53 54.03,11.22 IC1.16
N$70  (via drill 0.6)
  Top 0.305: 16.83,16.56 18.1,17.83 32.7,17.83 33.97,19.1 36.2,19.1 37.47,17.83 ISP1.3 | IC1.17 55.94,9.31 54.35,9.31 53.98,8.94 53.98,5.13 52.39,3.54 50.16,3.54 49.85,3.22 46.67,3.22 45.4,4.49 45.4,4.81 44.13,6.08 44.13,7.67 40.64,11.16 v32.7,11.16
  Top 0.406: R3.1 12.23,17.34 13.02,16.56 16.83,16.56
  Bottom 0.305: v32.7,11.16 32.7,17.83 33.81,18.94 36.04,18.94 37.47,17.51 ISP1.3
N$71
  Top 0.254: 63.56,16.82 63.88,16.82 64.14,16.56 64.45,16.56 64.77,16.24 70.48,16.24
  Top 0.305: IC1.32 63.56,16.82 | 70.48,16.24 71.44,15.29 87.31,15.29 89.22,13.38 IC16.8
N$72  (via drill 0.6)
  Top 0.305: IC10.10 63.5,37.83 v64.77,36.56 | v65.41,27.99 IC2.6
  Bottom 0.305: v64.77,36.56 64.77,28.62 v65.41,27.99
N$74
  Top 0.305: SV1.10 72.71,64.18 73.66,65.14 73.66,67.99 77.15,71.48 92.71,71.48 93.34,70.85 93.34,69.26 R6.2
N$76
  Top 0.305: IC16.2 73.98,9.57 73.34,8.94 69.22,8.94 67.94,10.21 62.55,10.21 61.91,10.84 60.96,10.84 60.64,10.53 60.64,9.82 IC1.23
N$77
  Top 0.305: IC16.3 76.52,9.57 75.25,8.3 68.9,8.3 67.63,9.57 61.69,9.57 IC1.24
N$78
  Top 0.305: IC1.25 66.42,11.22 67.94,12.75 78.74,12.75 79.06,12.43 IC16.4
N$79
  Top 0.305: IC1.26 66.26,12.02 67.63,13.38 80.96,13.38 81.6,12.75 IC16.5
N$80
  Top 0.305: IC1.27 66.11,12.82 67.31,14.02 83.5,14.02 84.14,13.38 IC16.6
N$81
  Top 0.305: IC1.28 65.64,13.62 66.67,14.65 85.72,14.65 86.68,13.7 IC16.7
N$82
  Top 0.254: C14.2 57.15,5.76 57.47,5.76 57.78,6.08 57.78,8.3 58.34,8.86 58.34,9.17
  Top 0.305: IC1.20 58.34,9.17
N$83  (via drill 0.6)
  Top 0.305: 33.02,16.07 R5.1 29.4,16.07 S1.2 S1.1 | 33.02,16.07 34.77,16.07 ISP1.5 | IC1.29 61.36,14.42 v60.96,14.02 | 32.63,15.68 33.02,16.07
  Bottom 0.406: v60.96,14.02 59.37,12.43 54.61,12.43 52.39,10.21 52.39,8.62 50.8,8.62 49.21,10.21 38.42,10.21 36.2,12.43 36.2,14.65 ISP1.5
N$84
  Top 0.305: IC1.7 56.74,19.51 56.52,19.73
  Top 0.406: C16.2 47.62,17.82 48.9,19.1 48.9,19.73 | 48.9,19.73 Q1.2 | 56.52,19.73 48.9,19.73
N$85
  Top 0.305: C15.2 49.09,12.43 Q1.1 50.48,13.83 50.48,16.88 51.92,18.31 IC1.8
N$86
  Top 0.305: SV1.8 75.56,64.18 76.2,64.82 76.2,68.63 77.79,70.22 88.58,70.22 R7.2
N$87
  Top 0.305: SV1.9 72.39,67.67 76.83,72.12 93.98,72.12 95.25,70.85 95.25,69.26 R8.1
N$88
  Top 0.305: SV1.7 74.93,68.31 77.47,70.85 91.44,70.85 92.08,70.22 92.08,69.26 R9.1
ROW_H_0
  Bottom 0.305: SV1.20 59.69,61.96 60.01,61.64 89.53,61.64 94.61,56.56 IC7.11
ROW_H_1
  Bottom 0.305: SV1.22 57.15,62.59 58.74,61.01 87.63,61.01 92.08,56.56 IC7.12
ROW_H_2
  Bottom 0.305: SV1.24 54.61,61.96 56.2,60.37 85.72,60.37 89.53,56.56 IC7.13
ROW_H_3
  Bottom 0.305: IC7.14 87,55.93 83.19,59.74 55.24,59.74 52.07,62.91 SV1.26
ROW_H_4
  Bottom 0.305: SV1.28 49.53,62.28 52.7,59.1 82.55,59.1 84.45,57.2 IC7.15
ROW_H_5
  Bottom 0.305: IC7.16 81.92,55.93 79.38,58.47 51.44,58.47 46.99,62.91 SV1.30
ROW_H_6
  Bottom 0.305: IC7.17 79.38,55.93 77.47,57.83 50.8,57.83 47.31,61.33 45.4,61.33 44.45,62.28 SV1.32
ROW_H_7
  Bottom 0.305: IC7.18 76.83,55.29 74.93,57.2 50.48,57.2 47.31,60.37 45.4,60.37 43.5,62.28 42.55,62.28 41.91,62.91 SV1.34
ROW_H_8
  Bottom 0.305: SV1.36 39.37,63.55 40.64,62.28 41.27,62.28 41.91,61.64 43.18,61.64 45.09,59.74 46.99,59.74 50.16,56.56 68.9,56.56 69.85,55.61 IC6.11
ROW_H_9
  Top 0.305: SV1.38 36.83,61.01 37.47,60.37 57.47,60.37 60.01,57.83 63.5,57.83 64.77,56.56 66.67,56.56 67.31,55.93 IC6.12
ROW_H_10
  Top 0.305: SV1.40 34.29,60.37 34.92,59.74 57.15,59.74 59.69,57.2 62.55,57.2 64.77,54.98 IC6.13
ROW_H_11
  Top 0.305: SV1.42 31.75,60.37 33.02,59.1 56.83,59.1 59.37,56.56 61.59,56.56 62.23,55.93 IC6.14
ROW_H_12
  Top 0.305: SV1.44 29.21,59.74 30.48,58.47 56.52,58.47 59.69,55.29 IC6.15
ROW_H_13
  Top 0.305: SV1.46 26.67,58.47 27.3,57.83 55.88,57.83 57.15,56.56 IC6.16
ROW_H_14
  Top 0.305: SV1.48 24.13,58.47 25.4,57.2 53.34,57.2 54.61,55.93 IC6.17
ROW_H_15
  Top 0.305: IC6.18 50.16,56.56 24.77,56.56 21.59,59.74 SV1.50
ROW_L_0
  Top 0.305: SV1.19 59.69,68.31 55.56,72.44 15.24,72.44 10.79,67.99 10.79,60.05 8.26,57.52 5.71,57.52 2.86,54.66 IC8.18
ROW_L_1
  Top 0.305: SV1.21 57.15,68.94 54.29,71.8 15.56,71.8 11.43,67.67 11.43,59.74 8.57,56.88 6.67,56.88 5.08,55.29 IC8.17
ROW_L_2
  Top 0.305: SV1.23 54.61,68.94 52.39,71.17 15.88,71.17 12.06,67.36 12.06,59.42 7.62,54.98 IC8.16
ROW_L_3
  Top 0.305: SV1.25 52.07,69.58 51.12,70.53 16.19,70.53 12.7,67.04 12.7,59.1 10.16,56.56 IC8.15
ROW_L_4
  Top 0.305: SV1.27 49.53,68.63 48.26,69.9 16.51,69.9 13.34,66.72 13.34,58.78 12.7,58.15 IC8.14
ROW_L_5
  Top 0.305: SV1.29 46.99,68.94 46.67,69.26 16.83,69.26 13.97,66.41 13.97,58.78 15.24,57.52 IC8.13
ROW_L_6
  Top 0.305: SV1.31 44.45,67.99 43.81,68.63 17.46,68.63 14.61,65.77 14.61,59.1 17.78,55.93 IC8.12
ROW_L_7
  Top 0.305: IC8.11 15.24,59.74 15.24,65.45 17.78,67.99 40.64,67.99 SV1.33
ROW_L_8
  Bottom 0.305: IC9.18 27.3,56.24 26.99,56.56 13.34,56.56 10.79,59.1 10.79,67.99 15.24,72.44 35.88,72.44 39.37,68.94 SV1.35
ROW_L_9
  Bottom 0.305: IC9.17 29.84,55.29 27.94,57.2 13.65,57.2 11.43,59.42 11.43,67.67 15.56,71.8 34.29,71.8 36.83,69.26 SV1.37
ROW_L_10
  Bottom 0.305: IC9.16 32.38,55.93 31.75,56.56 30.8,56.56 29.53,57.83 13.97,57.83 12.06,59.74 12.06,67.36 15.88,71.17 32.7,71.17 34.29,69.58 SV1.39
ROW_L_11
  Bottom 0.305: IC9.15 32.38,57.2 31.11,57.2 29.84,58.47 14.29,58.47 12.7,60.05 12.7,67.04 16.19,70.53 29.53,70.53 31.75,68.31 SV1.41
ROW_L_12
  Bottom 0.305: SV1.43 29.21,68.31 27.62,69.9 16.51,69.9 13.34,66.72 13.34,60.69 14.92,59.1 30.48,59.1 31.75,57.83 33.02,57.83 34.29,56.56 36.83,56.56 37.47,55.93 IC9.14
ROW_L_13
  Bottom 0.305: SV1.45 26.67,67.99 25.4,69.26 16.83,69.26 13.97,66.41 13.97,61.01 15.24,59.74 30.8,59.74 32.07,58.47 33.34,58.47 34.61,57.2 38.73,57.2 40.01,55.93 IC9.13
ROW_L_14
  Bottom 0.305: IC9.12 42.55,55.29 41.59,56.24 41.27,56.24 39.69,57.83 34.92,57.83 33.66,59.1 32.38,59.1 31.11,60.37 15.56,60.37 14.61,61.33 14.61,65.77 17.46,68.63 23.5,68.63 24.13,67.99 SV1.47
ROW_L_15
  Bottom 0.305: IC9.11 45.09,55.29 43.81,56.56 42.23,56.56 40.32,58.47 35.24,58.47 33.97,59.74 32.7,59.74 31.43,61.01 15.88,61.01 15.24,61.64 15.24,65.45 17.78,67.99 20.95,67.99 21.59,67.36 SV1.49
RX  (via drill 0.6, 0.7)
  Top 0.305: IC1.30 65.33,15.22 v65.41,15.29 | v55.24,6.08 55.24,4.49 55.56,4.17 66.99,4.17 JP1.3
  Bottom 0.305: v65.41,15.29 68.58,15.29 69.22,14.65 JP1.3 | v55.24,6.08 54.61,6.71 49.85,6.71 48.26,8.3 42.23,8.3 41.59,7.67 36.83,7.67 SV2.1
SR  (via drill 0.6)
  Top 0.305: IC4.6 18.73,23.54 23.5,19.1 32.07,19.1 34.29,21.32 34.29,22.27 | IC2.5 64.14,23.86 v65.09,22.91 | v78.74,23.23 IC3.4 | IC5.6 33.97,22.59 34.29,22.27 | 34.29,22.27 37.15,22.27 39.37,24.5 41.91,24.5 43.81,26.4 53.02,26.4 v54.93,24.5 | IC1.13 55.65,13.62 v56.2,13.38
  Bottom 0.305: v78.74,23.23 78.42,23.54 74.93,23.54 73.34,21.95 66.04,21.95 v65.09,22.91 | v54.93,24.5 55.88,24.5 | 55.88,24.5 57.47,24.5 58.42,23.54 64.45,23.54 v65.09,22.91 | v65.09,22.91 65.41,22.59 | v56.2,13.38 56.2,24.18 55.88,24.5
TX  (via drill 0.6, 0.7)
  Top 0.305: v60.96,15.61 61.59,15.61 61.91,15.92 62.94,15.92 IC1.31 | v55.56,2.91 56.2,2.91 56.83,3.54 68.26,3.54 70.48,5.76 70.48,7.35 70.17,7.67 67.31,7.67 66.67,7.03 JP1.2
  Bottom 0.305: JP1.2 66.67,12.43 63.5,15.61 v60.96,15.61 | v55.56,2.91 54.61,3.86 54.61,5.13 53.66,6.08 49.53,6.08 47.94,7.67 42.55,7.67 41.91,7.03 38.42,7.03 36.83,5.45 36.83,5.13 SV2.2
